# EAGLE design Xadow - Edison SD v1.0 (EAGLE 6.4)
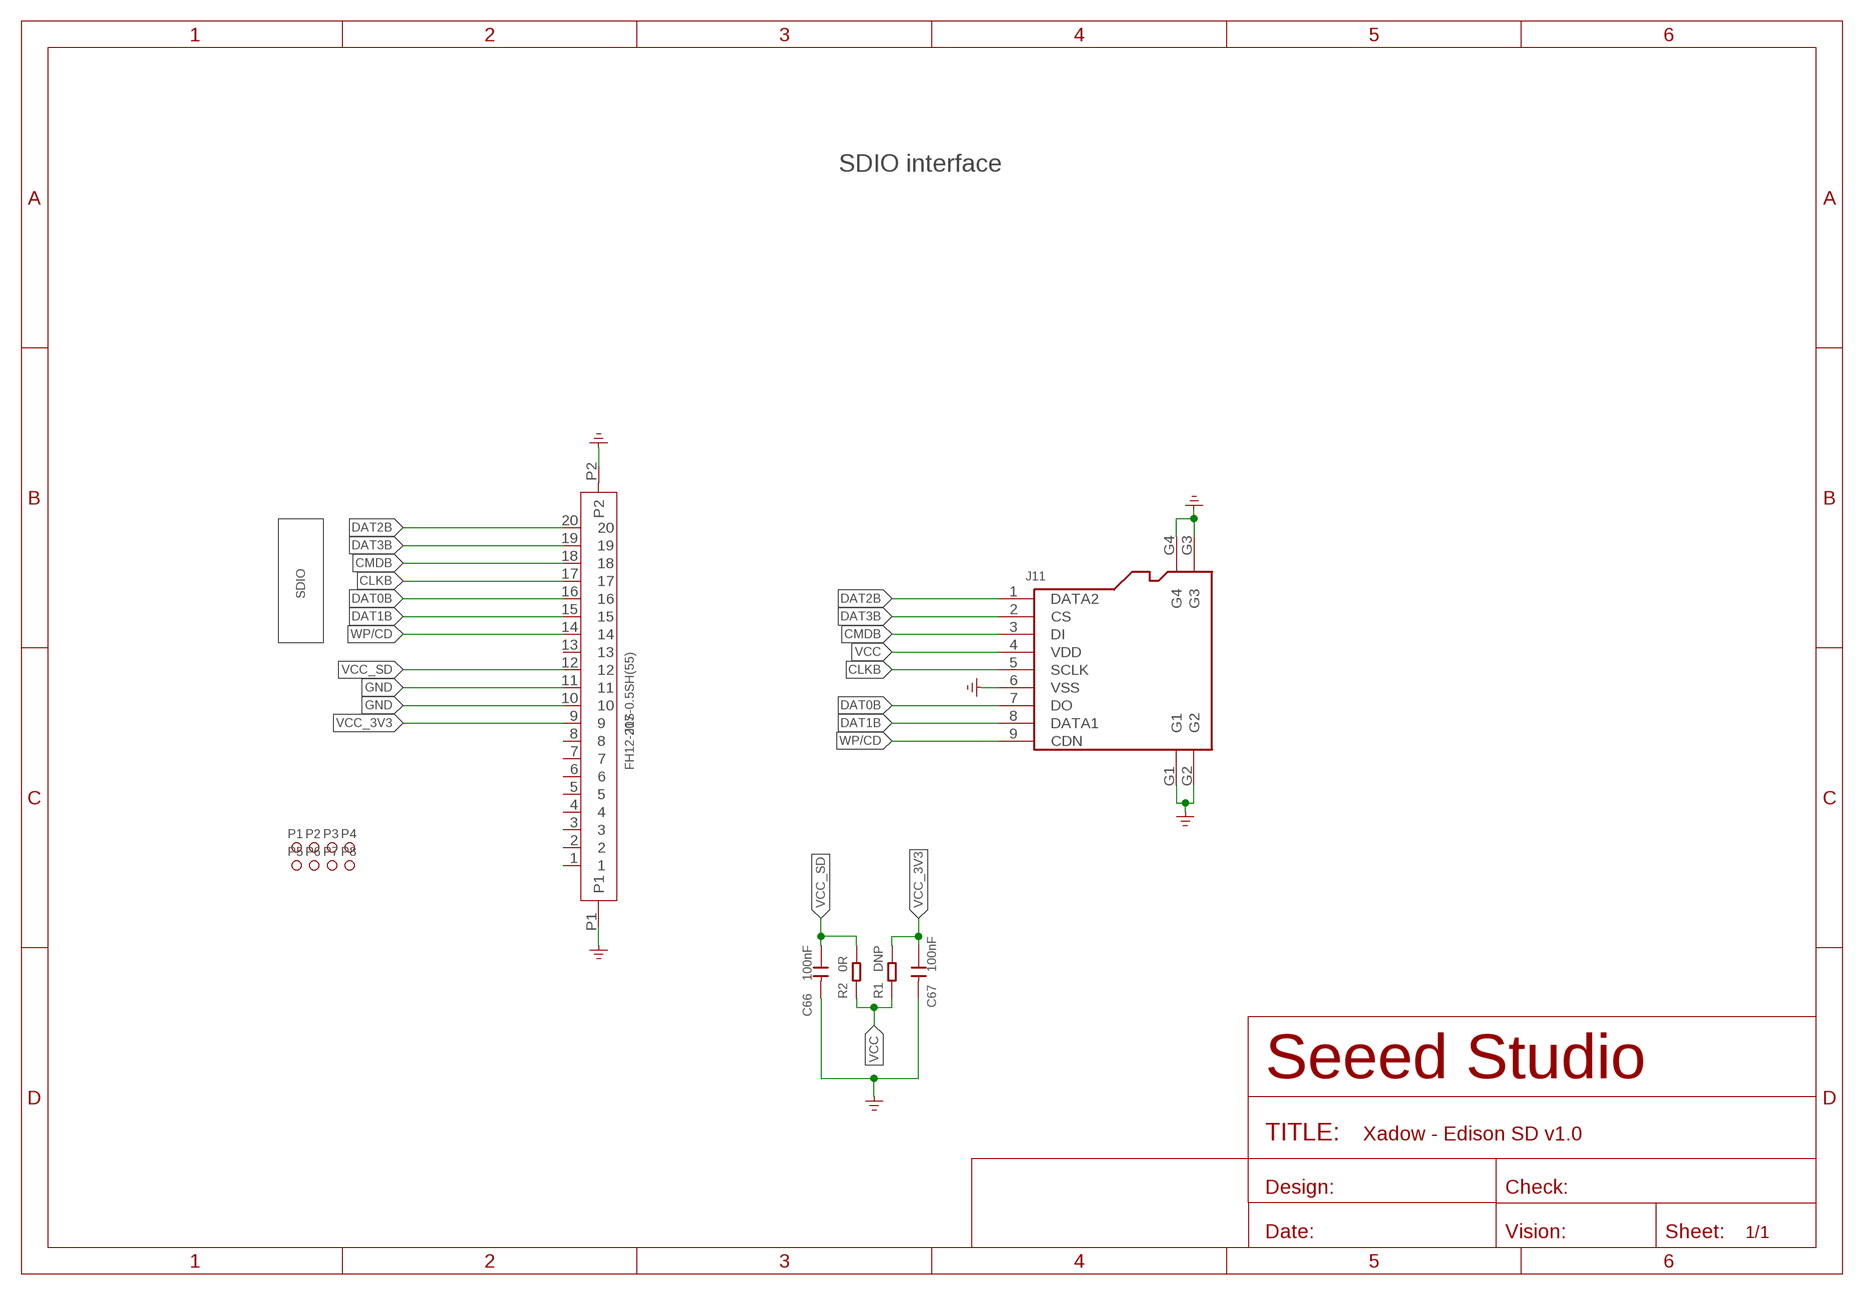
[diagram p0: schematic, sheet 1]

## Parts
C66  100nF  CAP-0402  [C0402]
C67  100nF  CAP-0402  [C0402]
J11  SD-CARD-MICRO-HOLDER-9P'MICROSD-9P'  [9+4P-SMD-L16.1*W14.5*H1.85MM]
J17  FH12-20S-0.5SH(55)  FH12-20S-0.5SH(55)FH12-20S-0.5SH  [20P-0.5]
P1  PAD-MARK'ANNULAR'  [ROUND-MARK-1.0]
P2  PAD-MARK'ANNULAR'  [ROUND-MARK-1.0]
P3  PAD-MARK'ANNULAR'  [ROUND-MARK-1.0]
P4  PAD-MARK'ANNULAR'  [ROUND-MARK-1.0]
P5  PAD-MARK'ANNULAR'  [ROUND-MARK-1.0]
P6  PAD-MARK'ANNULAR'  [ROUND-MARK-1.0]
P7  PAD-MARK'ANNULAR'  [ROUND-MARK-1.0]
P8  PAD-MARK'ANNULAR'  [ROUND-MARK-1.0]
R1  DNP  RES-0402  [R0402]
R2  0R  RES-0402  [R0402]

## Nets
CLKB: J11.5(SCLK) J17.17
CMDB: J11.3(DI) J17.18
DAT0B: J11.7(DO) J17.16
DAT1B: J11.8(DATA1) J17.15
DAT2B: J11.1(DATA2) J17.20
DAT3B: J11.2(CS) J17.19
GND: C66.2 C67.2 J11.6(VSS) J11.G1 J11.G2 J11.G3 J11.G4 J17.10 J17.11 J17.P1 J17.P2 ; supply symbol labelled GND_POWER
VCC: J11.4(VDD) R1.1 R2.1
VCC_3V3: C67.1 J17.9 R1.2
VCC_SD: C66.1 J17.12 R2.2
WP/CD: J11.9(CDN) J17.14
Unconnected: J17.1 J17.2 J17.3 J17.4 J17.5 J17.6 J17.7 J17.8 J17.13

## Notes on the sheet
- SDIO interface
- SDIO

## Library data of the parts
C66 C67 = Discrete-new:CAP: Ceramic Capacitors
J11 = Connector:SD-CARD-MICRO-HOLDER-9P: 320090008
J17 = template:FH12-20S-0.5SH(55)
P1-P8 = Discrete-new:PAD-MARK; PARTNO: DNP
R1 R2 = Discrete-new:RES

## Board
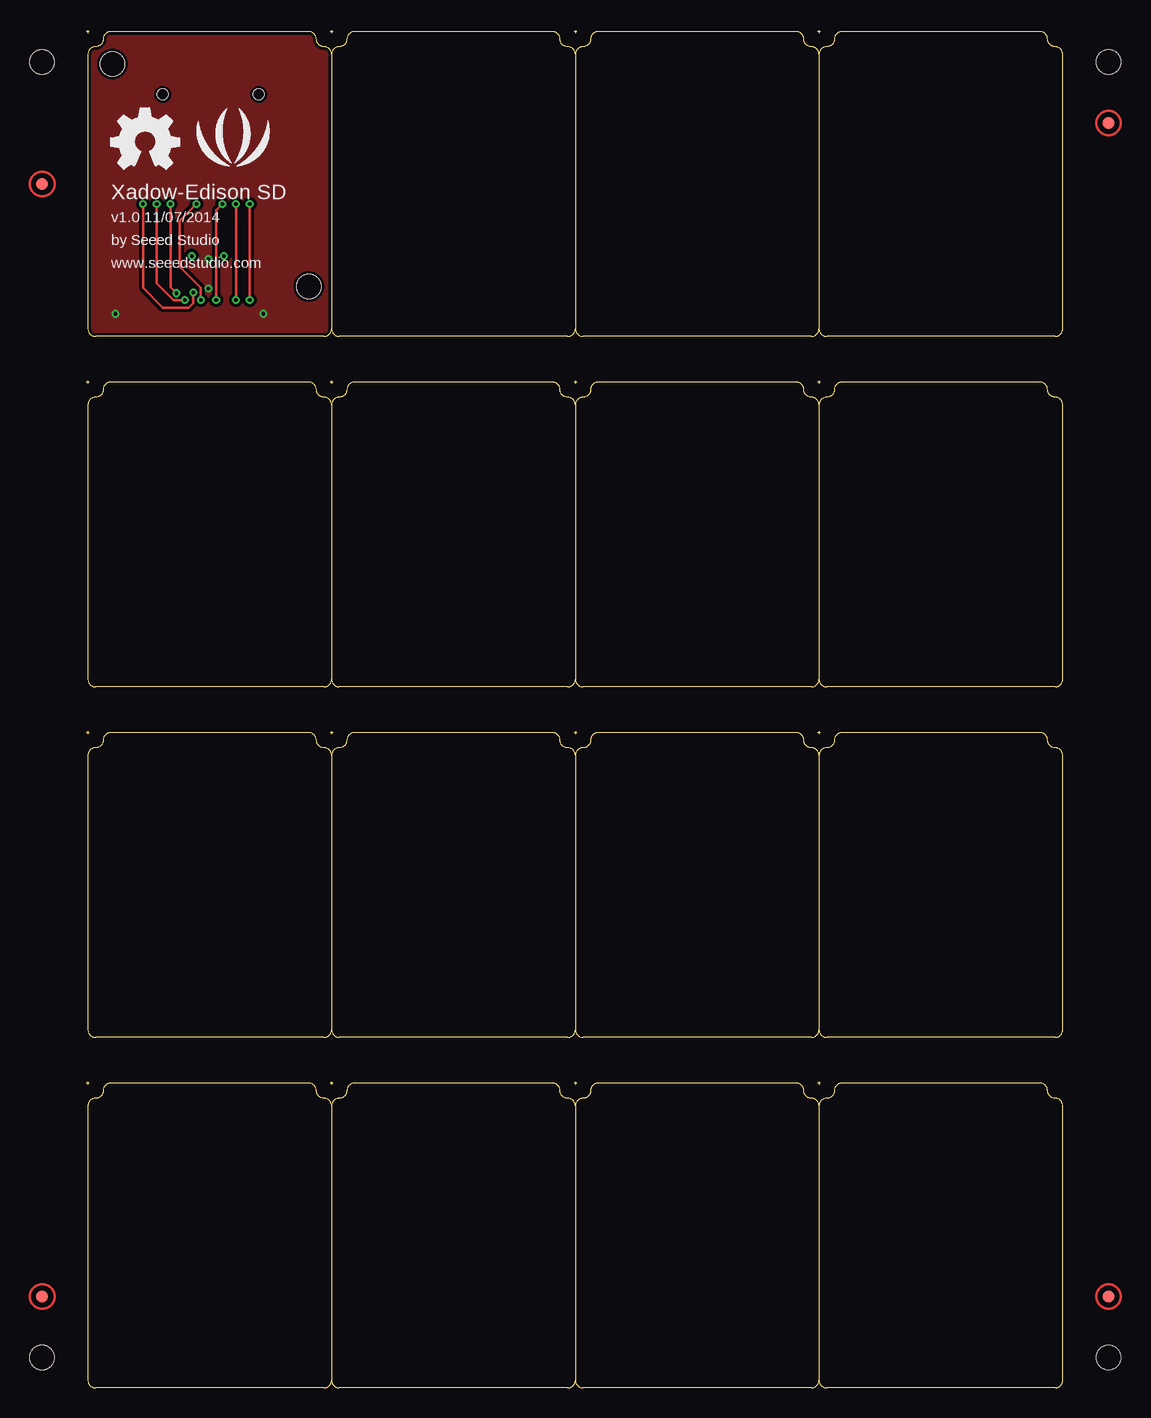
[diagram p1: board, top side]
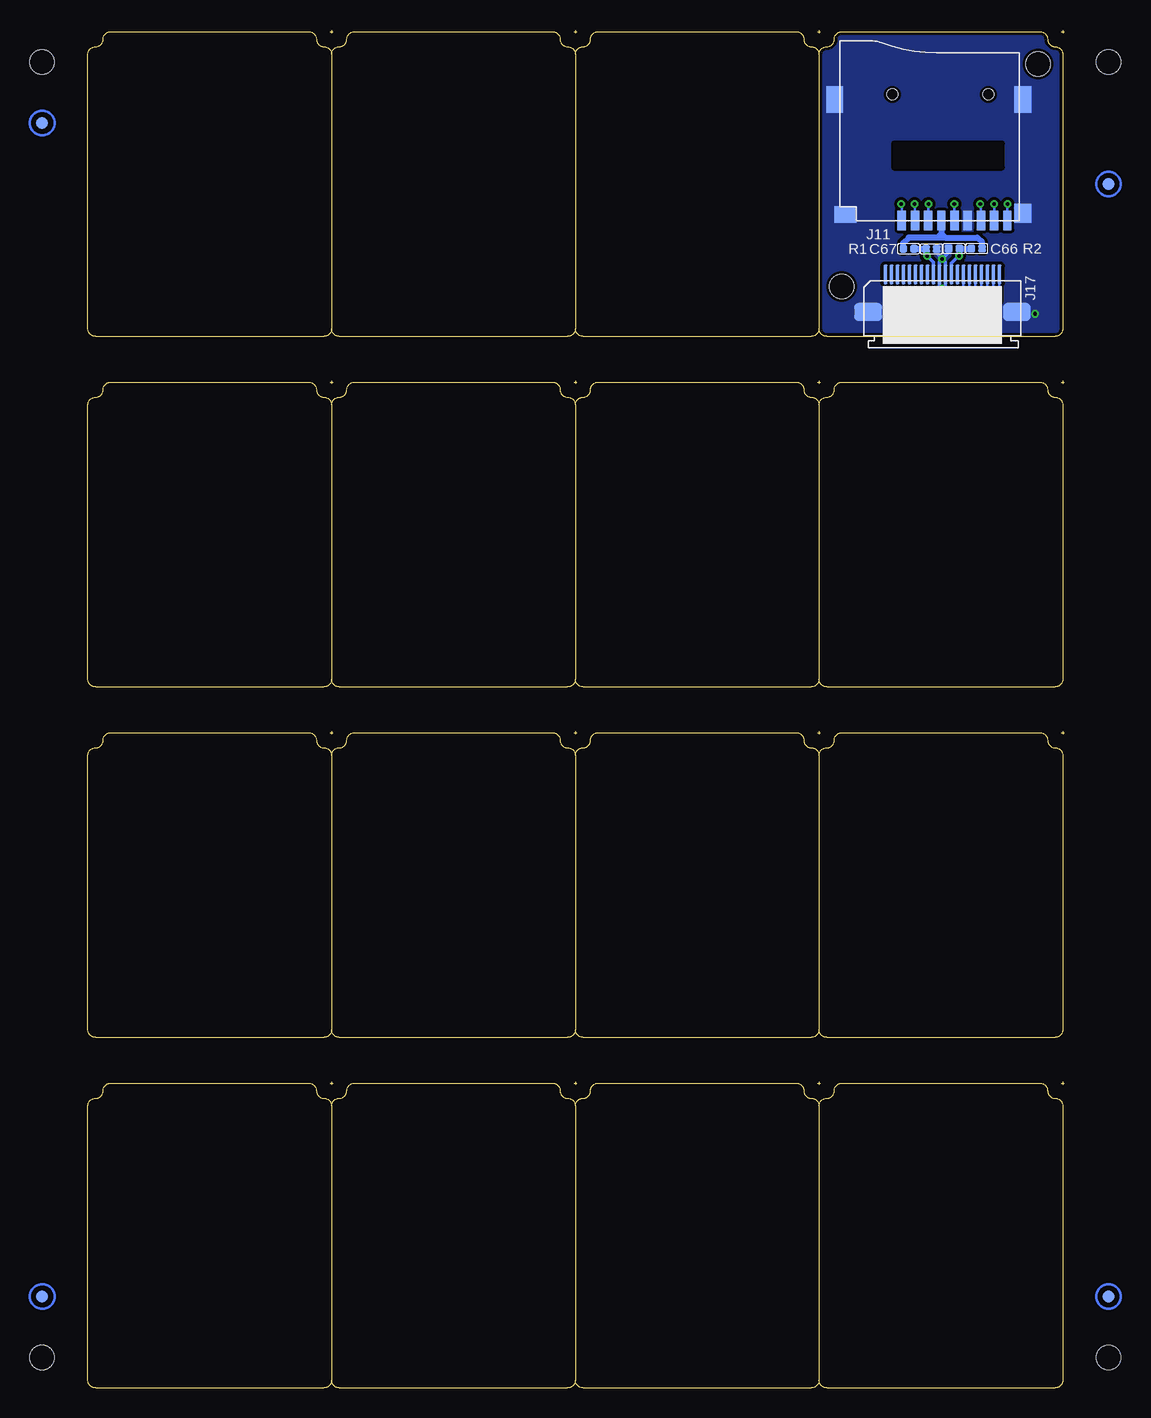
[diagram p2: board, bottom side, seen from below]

Size 81.41 x 113.16 mm. Coordinates in mm from the lower left corner, seen from the top.
Outline: 228 segments
Copper layers (1*16): Top 0.035mm / dielectric 1.5mm / Bottom 0.035mm
Design rules "SeeedStudio_2layer_DRU_no_angle_20140221 *": minimum track width 6mil, minimum drill 12mil, track to track 6mil, track to pad 6mil, pad to pad 6mil, via to via 6mil, smd to smd 0mil, copper to edge 10mil, drill to drill 10mil, minimum pad ring 10mil, minimum via ring 6mil, stop-mask expansion 2mil, vias tented up to drill 100mil, thermal gap 10mil
Holes 2.03 mm at 2.18,110.34 18.57,91.8 -3.68,110.49 85.22,110.49 -3.68,2.54 85.22,2.54

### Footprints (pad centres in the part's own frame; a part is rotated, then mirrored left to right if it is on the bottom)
C0402 = smd 0.635 x 0.635: 1 -0.445,0; 2 0.445,0
9+4P-SMD-L16.1*W14.5*H1.85MM = smd 1.6 x 0.7: 1 0,2.25; 2 0,1.15; 3 0,0.05; 4 0,-1.05; 5 0,-2.15; 6 0,-3.25; 7 0,-4.35; 8 0,-5.45; 9 0,-6.55 | smd 1.6 x 1.4: G1 0.6,-7.85 | smd 2.2 x 1.4: G2 10.1,-7.85; G3 10.1,7.85 | smd 1.4 x 1.8: G4 0.5,6.95 | hole 0.9: 10.5,-4.95; 10.5,3.05
20P-0.5 = smd 0.3 x 1.6: 1 -4.75,3.127; 2 -4.25,3.127; 3 -3.75,3.127; 4 -3.25,3.127; 5 -2.75,3.127; 6 -2.25,3.127; 7 -1.75,3.127; 8 -1.25,3.127; 9 -0.75,3.127; 10 -0.25,3.127; 11 0.25,3.127; 12 0.75,3.127; 13 1.25,3.127; 14 1.75,3.127; 15 2.25,3.127; 16 2.75,3.127; 17 3.25,3.127; 18 3.75,3.127; 19 4.25,3.127; 20 4.75,3.127 | smd 2.3 x 1.5: P1 -6.2,0; P2 6.2,0
ROUND-MARK-1.0 = smd 1.016 x 1.016: P$1 0,0
R0402 = smd 0.635 x 0.635: 1 -0.445,0; 2 0.445,0

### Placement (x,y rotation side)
C66  9.19,94.95 180 bottom
C67  11.09,94.92 0 bottom
J11  11.3,97.28 90 bottom
J17  10.16,89.66 0 bottom
P1  not placed on the board
P2  not placed on the board
P3  not placed on the board
P4  not placed on the board
P5  not placed on the board
P6  not placed on the board
P7  not placed on the board
P8  not placed on the board
R1  12.98,94.93 0 bottom
R2  7.3,94.95 180 bottom
U$40  [LOGO_SILK]  12.22,103.48 0 top
U$63  [OSHW_FILLX200_NOTEXT]  2.06,101.57 0 top

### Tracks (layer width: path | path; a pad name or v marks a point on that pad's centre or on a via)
CLKB  (via drill 0.3 pad 0.64)
  Top 0.203: v9.55,90.65 9.55,91.67 7.77,93.45 7.77,97.26 v9.17,98.65
  Bottom 0.203: J17.17 6.91,90.81 7.7,90.02 8.92,90.02 v9.55,90.65 | J11.5 9.15,98.64 v9.17,98.65
CMDB  (via drill 0.3 pad 0.64)
  Top 0.203: v10.82,90.65 10.82,98.15 v11.33,98.65
  Bottom 0.203: J17.18 6.41,90.7 7.47,89.64 9.8,89.64 v10.82,90.65 | J11.3 11.35,98.63 v11.33,98.65
DAT0B  (via drill 0.3 pad 0.64)
  Top 0.203: v7.01,98.65 7.01,91.73 v7.52,91.22
  Bottom 0.203: J11.7 6.95,98.6 v7.01,98.65 | J17.16 7.41,91.33 v7.52,91.22
DAT1B  (via drill 0.3 pad 0.64)
  Top 0.203: v8.22,90.65 7.26,90.65 5.87,92.05 v5.87,98.65
  Bottom 0.203: J11.8 5.85,98.64 v5.87,98.65 | J17.15 7.91,91.66 8.22,91.35 v8.22,90.65
DAT2B  (via drill 0.3 pad 0.64)
  Top 0.203: v13.61,90.65 v13.61,98.65
  Bottom 0.203: J17.20 5.41,90.54 7.2,88.75 11.71,88.75 v13.61,90.65 | J11.1 13.55,98.59 v13.61,98.65
DAT3B  (via drill 0.3 pad 0.64)
  Top 0.203: v12.47,90.65 v12.47,98.65
  Bottom 0.203: J17.19 5.91,90.59 7.25,89.26 11.07,89.26 v12.47,90.65 | J11.2 12.45,98.64 v12.47,98.65
GND  (via drill 0.3 pad 0.64)
  Bottom 0.305: v10.19,94.08 10.41,93.86 J17.10 10.41,91.77 10.19,91.54 | v10.19,94.08 9.91,93.81 J17.11 9.91,91.82 10.19,91.54 | 10.19,91.54 v10.19,91.61 | C66.2 9.64,94.63 v10.19,94.08 | C67.2 10.64,94.54 v10.19,94.08
  other vias: 14.76,89.51 2.44,89.51
  pour Bottom (isolate 0.254, rank 6, no thermals): -0.61,113.51 20.98,113.51 20.98,86.84 -0.61,86.84
  pour Top (isolate 0.254, rank 6, no thermals): -0.61,113.51 20.98,113.51 20.98,86.84 -0.61,86.84
VCC
  Bottom 0.508: 9.93,95.86 10.19,95.86 | 10.19,95.86 10.57,95.86 | J11.4 10.25,96.18 | 10.25,96.17 10.25,95.93 10.19,95.86 | 10.25,96.18 9.93,95.86 | 10.25,96.18 10.25,96.17 | 10.25,96.17 10.57,95.86 | 9.93,95.86 7.26,95.86 6.86,95.45 R2.1 | 10.57,95.86 12.98,95.86 13.42,95.42 R1.1
VCC_3V3  (via drill 0.3 pad 0.64)
  Bottom 0.305: J17.9 10.91,93.79 v11.46,94.34
  Bottom 0.508: C67.1 11.53,94.84 | 11.53,94.84 11.53,94.41 v11.46,94.34 | R1.2 11.62,94.93 11.53,94.84
VCC_SD  (via drill 0.3 pad 0.64)
  Bottom 0.305: J17.12 9.41,93.71 v8.79,94.34
  Bottom 0.508: v8.79,94.34 8.75,94.37 C66.1 R2.2
WP/CD  (via drill 0.3 pad 0.64)
  Top 0.203: v8.92,91.29 8.92,90.4 8.53,90.02 6.38,90.02 4.72,91.67 v4.72,98.65
  Bottom 0.203: J17.14 8.41,91.79 v8.92,91.29 | J11.9 4.75,98.62 v4.72,98.65

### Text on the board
tPlace: Xadow-Edison SD | v1.0 11/07/2014 | by Seeed Studio | www.seeedstudio.com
